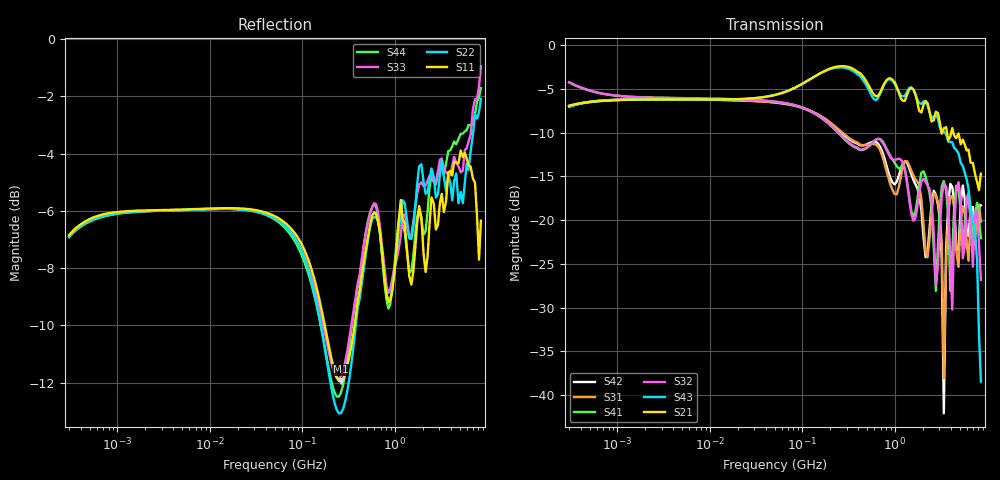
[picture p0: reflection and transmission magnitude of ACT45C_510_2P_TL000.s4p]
! S-Parameter Data Generated by TDK Corporation
! Copyright(C) 2025 TDK Corporation.
! All Rights Reserved.
! TDK P/N: ACT45C-510-2P-TL000 (Signal Line Common Mode Choke/Filter)
! Property: |Zc|=2800ohm at 10MHz
! Size(LxWxT): 4.5x3.2x2.8mm
! Model Type: s2p (Touchstone File Format Version 1.0)
! Frequency: DC=Yes Start=0.3MHz Stop=8500MHz 202points Log-sweep
! Model Generated on July 30, 2025
! Terms and conditions regarding TDK Simulation Models:
! 1)This simulation model is being provided solely for informational
!  purposes. Please refer to the specifications of the products in
!  terms of detailed characteristics of such products.
! 2)In no event shall TDK Corporation of any of its subsidiaries be
!  liable for any loss or damage arising, directly or indirectly,
!  from any information contained in this simulation model, including,
!  but not limited to loss or damages arising from any inaccuracies,
!  omissions or errors in connection with such information.
! 3)Any and all copyrights on this simulation model are owned by
!  TDK Corporation.  Duplication or redistribution of this simulation
!  model without prior written permission from TDK Corporation
!  is prohibited.
! 4)This simulation model is subject to any modification or change
!  without any prior notice.
! 5)Neither TDK Corporation nor any of its subsidiaries shall make any
!  warranty, express or implied, including but not limited to the
!  correctness, implied warranties of merchantability and fitness for
!  a particular purpose with respect to this simulation models.
! 6)The use of this simulation model shall be deemed to have consented
!  to the terms and conditions hereof.
! Port Assignments:
!  1 ---@@@--- 4
!  2 ---@@@--- 3
! Applicable Conditions:
!  Temperature = 25 degC
!  DC Bias Current = 0 A
!  Small Signal Operation
# Hz S MA R 50
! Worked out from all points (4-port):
!   201 points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, 300 kHz to 8.5 GHz, reference 50 ohm
!   strongest paths, dB at 300 kHz, 3.892 MHz, 50.5 MHz, 655.2 MHz, 8.5 GHz:
!     S21: -6.9, -6.2, -5.7, -5.8, -14.7
!     S43: -7.0, -6.2, -5.7, -6.1, -38.5
!     S32: -4.2, -6.0, -6.4, -10.7, -26.8
!     S41: -4.2, -6.0, -6.5, -10.7, -22.1
!     S31: -6.9, -6.2, -6.5, -11.6, -20.2
!     S42: -7.0, -6.2, -6.5, -11.2, -18.3
!   lowest |S11| = -12.0 dB at 260.4 MHz (marker M1), VSWR 1.68, Z = 83.6 - j2.73 ohm
!   |S11| at or under -10 dB: 174.5 MHz to 366.3 MHz (191.8 MHz wide, 70.9 % of centre)
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300000  0.4551 23.8  0.4504 24.4  0.4491 -155.9  0.6166 -17.3
        0.4514 24.5  0.452 23.7  0.6161 -18.0  0.4506 -155.1
        0.4501 -155.3  0.6148 -17.5  0.4528 23.9  0.45 25.6
        0.6131 -17.6  0.4457 -155.3  0.4466 24.8  0.4509 25.0
2.60398e8  0.2525 -3.5  0.7594 -6.5  0.3204 78.0  0.3028 -104.4
           0.7594 -6.6  0.2221 0.0  0.3063 -103.6  0.3157 73.6
           0.3215 77.9  0.3062 -103.6  0.2578 2.2  0.7468 -8.6
           0.3044 -104.4  0.3163 73.7  0.7468 -8.6  0.2411 4.1
2.77421e9  0.4652 -54.0  0.4165 -55.1  0.1379 32.5  0.03958 176.1
           0.417 -56.0  0.5289 -50.5  0.03795 -141.7  0.141 37.4
           0.1397 31.1  0.04284 -139.1  0.562 -41.7  0.3943 -73.7
           0.03938 174.2  0.1396 36.1  0.4011 -73.3  0.5575 -45.8
3.378408e9  0.499 -59.8  0.3372 -62.9  0.01107 -115.1  0.1676 20.2
            0.3352 -61.4  0.5757 -59.9  0.1605 44.7  0.007759 158.7
            0.01248 -113.1  0.1616 43.9  0.5956 -52.8  0.3214 -83.0
            0.1674 19.9  0.007867 157.5  0.322 -83.3  0.5803 -54.3
3.970576e9  0.5882 -68.1  0.3003 -65.9  0.1382 17.6  0.03846 -32.0
            0.3007 -65.5  0.5603 -71.0  0.05795 -44.8  0.1579 19.9
            0.1363 17.8  0.05938 -42.7  0.5782 -59.3  0.2855 -92.4
            0.03943 -32.6  0.1612 19.7  0.2799 -93.4  0.6401 -63.3
7.34696e9  0.5613 -145.8  0.1833 -141.9  0.0741 -117.3  0.1141 -89.8
           0.1838 -141.8  0.7391 -125.1  0.09955 -61.6  0.08678 -90.8
           0.07997 -112.2  0.1088 -57.5  0.7857 -120.7  0.08343 172.0
           0.1091 -85.5  0.08252 -86.8  0.08699 169.5  0.7402 -134.1
8.5e9  0.4817 -152.0  0.1844 -147.9  0.09084 -157.0  0.0818 -124.4
       0.1845 -148.1  0.7866 -92.8  0.04196 -61.7  0.1255 -89.7
       0.09822 -146.7  0.04562 -51.8  0.8971 -95.1  0.01193 102.0
       0.07891 -115.8  0.1216 -80.7  0.01195 95.5  0.8216 -131.8
